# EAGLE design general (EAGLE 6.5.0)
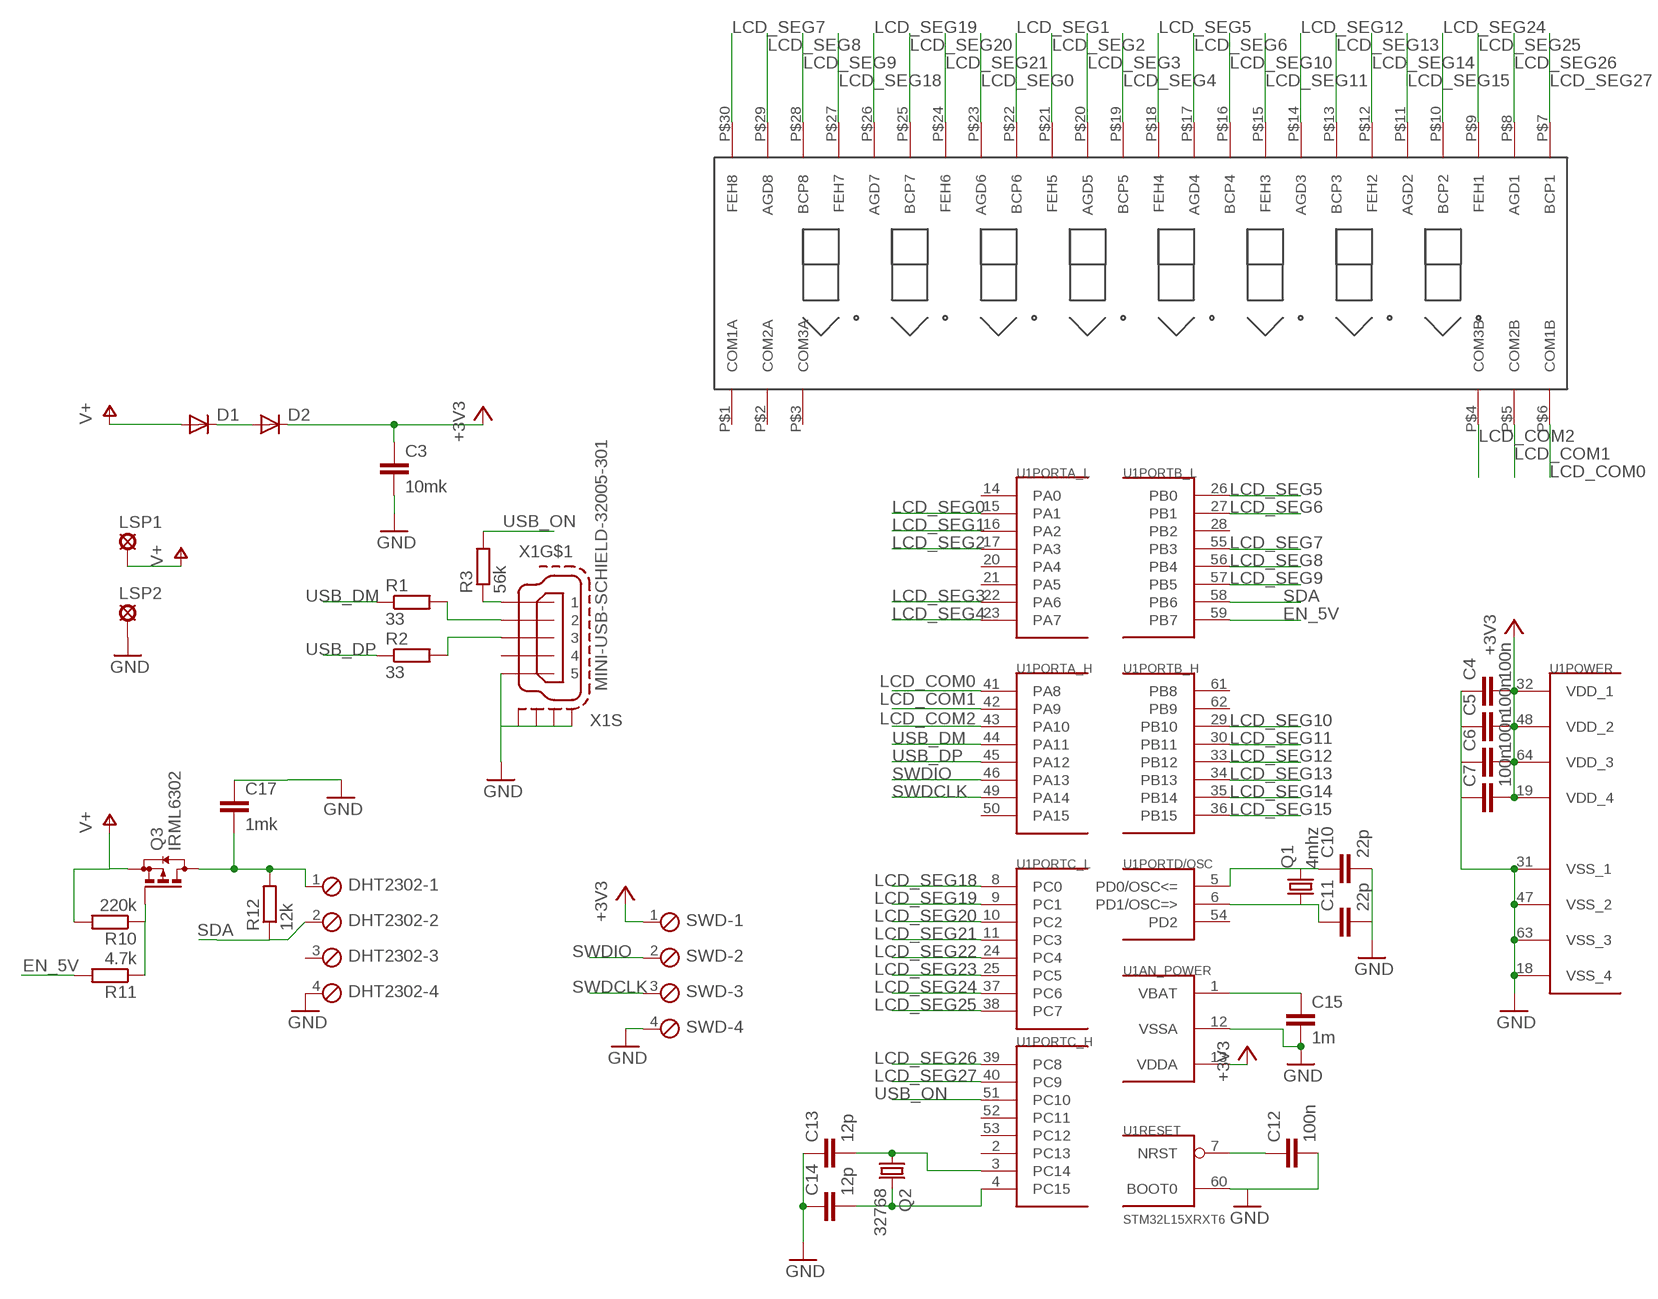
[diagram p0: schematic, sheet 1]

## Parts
C3  10mk  C-EUC0805  [C0805]
C4  100n  C-EUC0603  [C0603]
C5  100n  C-EUC0603  [C0603]
C6  100n  C-EUC0603  [C0603]
C7  100n  C-EUC0603  [C0603]
C10  22p  C-EUC0603  [C0603]
C11  22p  C-EUC0603  [C0603]
C12  100n  C-EUC0603  [C0603]
C13  12p  C-EUC0805  [C0805]
C14  12p  C-EUC0805  [C0805]
C15  1m  C-EUC0603  [C0603]
C17  1mk  C-EUC0603  [C0603]
D1  CGRM4004-G  [SOD-123_MINI-SMA]
D2  CGRM4004-G  [SOD-123_MINI-SMA]
DHT2302  MPT4  [4POL254]
LSP1  SE14  [SE14]
LSP2  SE14  [SE14]
Q1  4mhz  CRYSTALHC49S  [HC49/S]
Q2  32768  CRYSTALTC26H  [TC26H]
Q3  IRML6302  BSS84  [SOT23]
R1  33  R-EU_M0805  [M0805]
R2  33  R-EU_M0805  [M0805]
R3  56k  R-EU_R0805  [R0805]
R10  220k  R-EU_R0805  [R0805]
R11  4.7k  R-EU_R0805  [R0805]
R12  12k  R-EU_R0805  [R0805]
SWD  MPT4  [4POL254]
U1  STM32L15XRXT6  STM32F10XRXT6  [TQFP64]
U$1  TI8077  [TI8077]
X1  MINI-USB-SCHIELD-32005-301  [32005-301]

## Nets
+3V3: C3.1 C4.2 C5.2 C6.2 C7.2 D2.C SWD.1 U1.13(AN_POWER:VDDA) U1.19(POWER:VDD_4) U1.32(POWER:VDD_1) U1.48(POWER:VDD_2) U1.64(POWER:VDD_3)
+5V: D1.A LSP1.MP Q3.2(S) R10.2 ; supply symbol labelled V+
EN_5V: R11.2 U1.59(PORTB_L:PB7)
GND: C3.2 C4.1 C5.1 C6.1 C7.1 C10.2 C11.2 C12.2 C13.1 C14.1 C15.2 C17.1 DHT2302.4 LSP2.MP SWD.4 U1.12(AN_POWER:VSSA) U1.18(POWER:VSS_4) U1.31(POWER:VSS_1) U1.47(POWER:VSS_2) U1.60(RESET:BOOT0) U1.63(POWER:VSS_3) X1.5 X1.M1(S:S1) X1.M2(S:S2) X1.M3(S:S3) X1.M4(S:S4)
LCD_COM0: U1.41(PORTA_H:PA8) U$1.P$6(COM1B)
LCD_COM1: U1.42(PORTA_H:PA9) U$1.P$5(COM2B)
LCD_COM2: U1.43(PORTA_H:PA10) U$1.P$4(COM3B)
LCD_SEG0: U1.15(PORTA_L:PA1) U$1.P$23(AGD6)
LCD_SEG1: U1.16(PORTA_L:PA2) U$1.P$22(BCP6)
LCD_SEG2: U1.17(PORTA_L:PA3) U$1.P$21(FEH5)
LCD_SEG3: U1.22(PORTA_L:PA6) U$1.P$20(AGD5)
LCD_SEG4: U1.23(PORTA_L:PA7) U$1.P$19(BCP5)
LCD_SEG5: U1.26(PORTB_L:PB0) U$1.P$18(FEH4)
LCD_SEG6: U1.27(PORTB_L:PB1) U$1.P$17(AGD4)
LCD_SEG7: U1.55(PORTB_L:PB3) U$1.P$30(FEH8)
LCD_SEG8: U1.56(PORTB_L:PB4) U$1.P$29(AGD8)
LCD_SEG9: U1.57(PORTB_L:PB5) U$1.P$28(BCP8)
LCD_SEG10: U1.29(PORTB_H:PB10) U$1.P$16(BCP4)
LCD_SEG11: U1.30(PORTB_H:PB11) U$1.P$15(FEH3)
LCD_SEG12: U1.33(PORTB_H:PB12) U$1.P$14(AGD3)
LCD_SEG13: U1.34(PORTB_H:PB13) U$1.P$13(BCP3)
LCD_SEG14: U1.35(PORTB_H:PB14) U$1.P$12(FEH2)
LCD_SEG15: U1.36(PORTB_H:PB15) U$1.P$11(AGD2)
LCD_SEG18: U1.8(PORTC_L:PC0) U$1.P$27(FEH7)
LCD_SEG19: U1.9(PORTC_L:PC1) U$1.P$26(AGD7)
LCD_SEG20: U1.10(PORTC_L:PC2) U$1.P$25(BCP7)
LCD_SEG21: U1.11(PORTC_L:PC3) U$1.P$24(FEH6)
LCD_SEG22: U1.24(PORTC_L:PC4)
LCD_SEG23: U1.25(PORTC_L:PC5)
LCD_SEG24: U1.37(PORTC_L:PC6) U$1.P$10(BCP2)
LCD_SEG25: U1.38(PORTC_L:PC7) U$1.P$9(FEH1)
LCD_SEG26: U1.39(PORTC_H:PC8) U$1.P$8(AGD1)
LCD_SEG27: U1.40(PORTC_H:PC9) U$1.P$7(BCP1)
N$1: R1.2 X1.2
N$2: R2.2 X1.3
N$3: D1.C D2.A
N$9: C14.2 Q2.2 U1.4(PORTC_H:PC15)
N$10: Q3.1(G) R10.1 R11.1
N$11: R3.1 X1.1
N$13: C15.1 U1.1(AN_POWER:VBAT)
N$33: C10.1 Q1.2 U1.5(PORTD/OSC:PD0/OSC<=)
N$34: C11.1 Q1.1 U1.6(PORTD/OSC:PD1/OSC=>)
N$35: C13.2 Q2.1 U1.3(PORTC_H:PC14)
N$36: C12.1 U1.7(RESET:NRST)
SDA: DHT2302.2 R12.1 U1.58(PORTB_L:PB6)
STABILIZE_5V: C17.2 DHT2302.1 Q3.3(D) R12.2
SWDCLK: SWD.3 U1.49(PORTA_H:PA14)
SWDIO: SWD.2 U1.46(PORTA_H:PA13)
USB_DM: R1.1 U1.44(PORTA_H:PA11)
USB_DP: R2.1 U1.45(PORTA_H:PA12)
USB_ON: R3.2 U1.51(PORTC_H:PC10)
Unconnected: DHT2302.3 U1.2(PORTC_H:PC13) U1.14(PORTA_L:PA0) U1.20(PORTA_L:PA4) U1.21(PORTA_L:PA5) U1.28(PORTB_L:PB2) U1.50(PORTA_H:PA15) U1.52(PORTC_H:PC11) U1.53(PORTC_H:PC12) U1.54(PORTD/OSC:PD2) U1.61(PORTB_H:PB8) U1.62(PORTB_H:PB9) U$1.P$1(COM1A) U$1.P$2(COM2A) U$1.P$3(COM3A) X1.4

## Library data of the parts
C3-C7 C10-C12 C15 C17 = rcl:C-EU: CAPACITOR, European symbol
C13 C14 = resistor:C-EU: CAPACITOR, European symbol
D1 D2 = diode:CGRM400*-G: Molded plasitc,JEDEC SOD-123/Mini SMA
DHT2302 SWD = con-phoenix-254:MPT4: PHOENIX CONNECTOR; OC_FARNELL: unknown; OC_NEWARK: unknown
LSP1 LSP2 = solpad:SE14: SOLDER PAD
Q1 = crystal:CRYSTAL: CRYSTAL; OC_FARNELL: 1667008; OC_NEWARK: unknown
Q2 = crystal:CRYSTAL: CRYSTAL; OC_FARNELL: unknown; OC_NEWARK: unknown
Q3 = transistor-small-signal:BSS84: P-CHANNEL MOS FET
R1-R3 R10-R12 = rcl:R-EU_: RESISTOR, European symbol
U1 = stm32:STM32F10XRXT6: STM32F101/103 64pin LQFP
U$1 = balmer:TI8077: LCD Display
X1 = con-cypressindustries:MINI-USB-SCHIELD-: MINI USB-B Conector Source: www.cypressindustries.com; OC_FARNELL: unknown; OC_NEWARK: unknown

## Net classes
0 default: clearance 0.15 mm

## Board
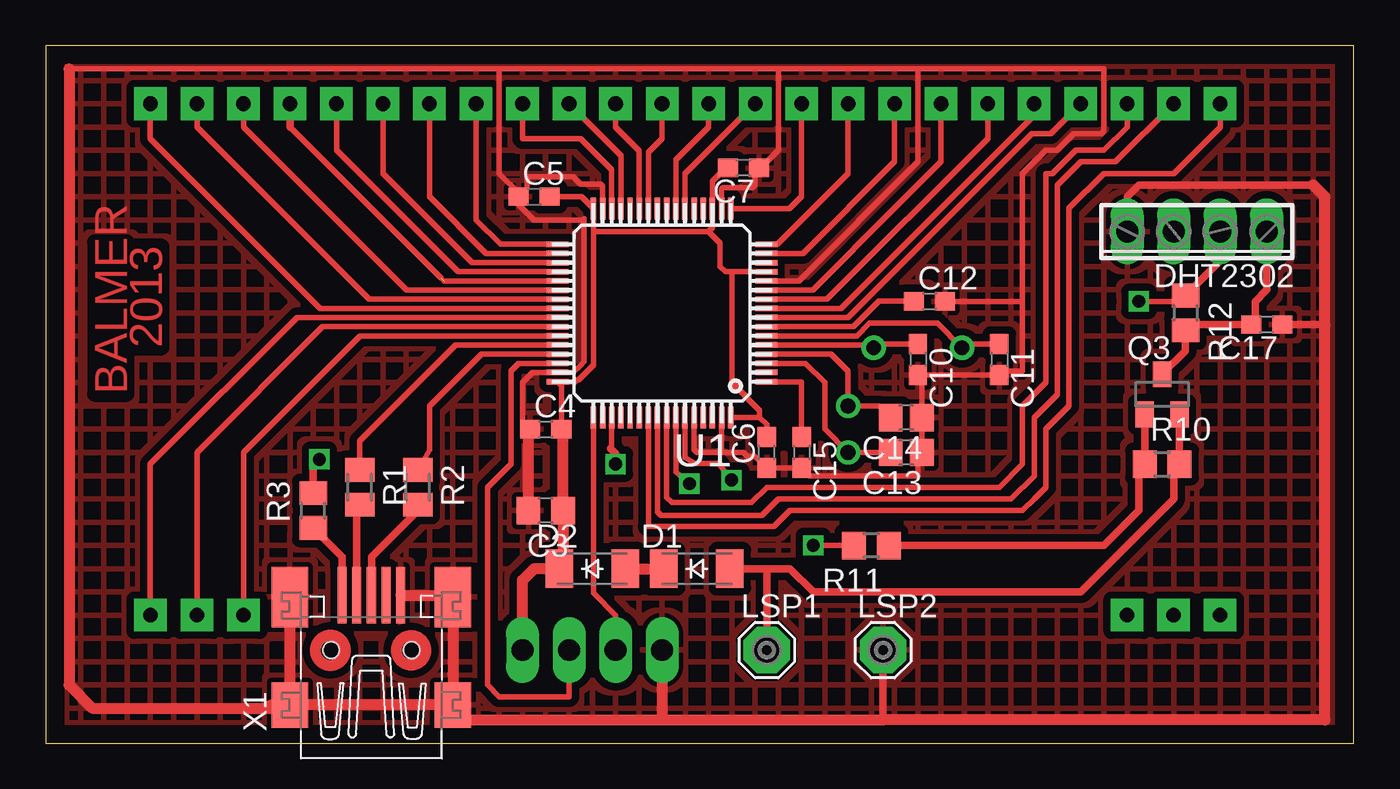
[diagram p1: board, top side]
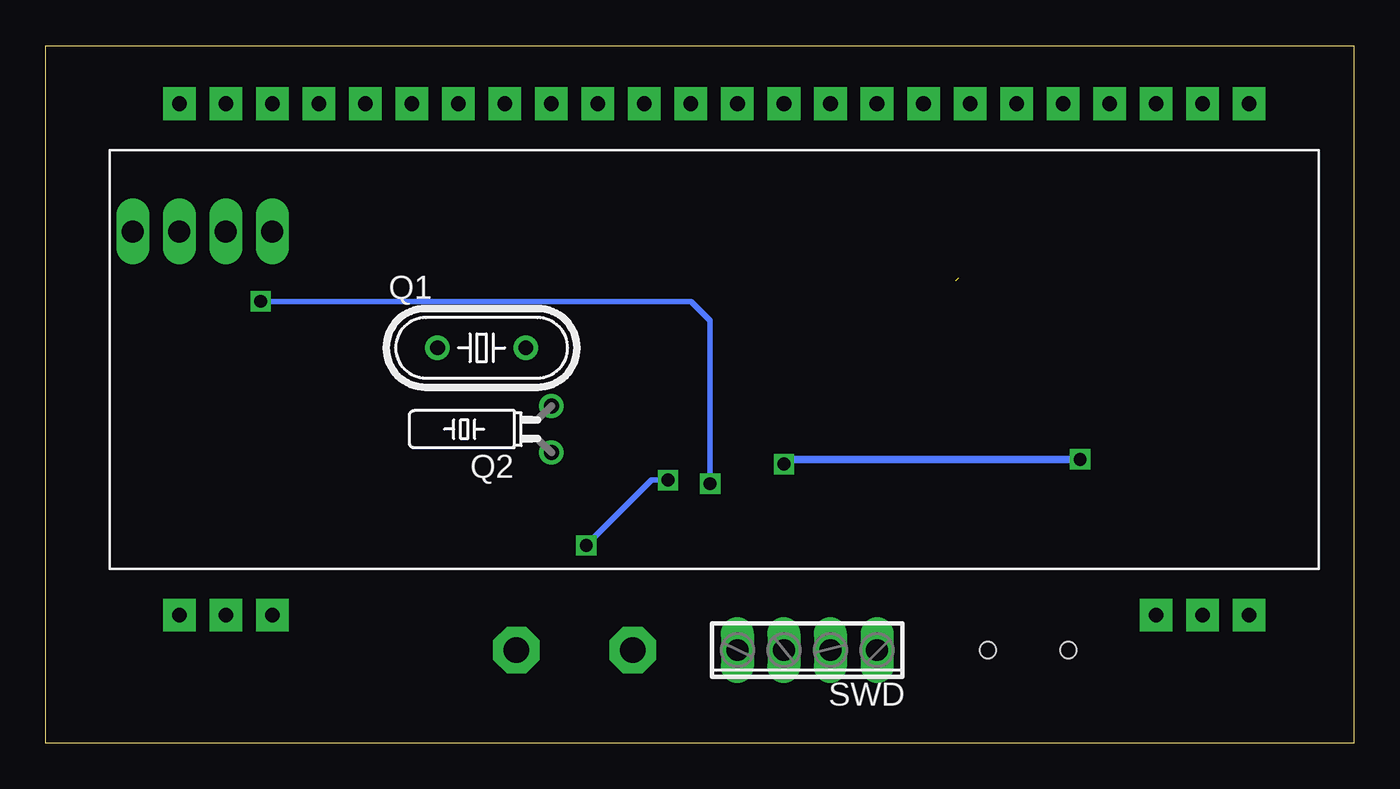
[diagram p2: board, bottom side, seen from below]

Size 71.43 x 38.09 mm. Coordinates in mm from the lower left corner, seen from the top.
Outline: 0,0 71.43,0 71.43,38.09 0,38.09 0,0
Copper layers (1*16): Top 0.035mm / dielectric 1.5mm / Bottom 0.035mm
Design rules "default": minimum track width 10mil, minimum drill 24mil, track to track 8mil, track to pad 8mil, pad to pad 8mil, via to via 8mil, smd to smd 8mil, copper to edge 40mil, drill to drill 8mil, minimum pad ring 10mil, minimum via ring 8mil, stop-mask expansion 4mil, vias tented up to drill 0mil, thermal gap 10mil

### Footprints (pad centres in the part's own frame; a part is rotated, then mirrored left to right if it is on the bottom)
C0805 = smd 1.3 x 1.5: 1 -0.95,0; 2 0.95,0
C0603 = smd 1.1 x 1: 1 -0.85,0; 2 0.85,0
C0805' = smd 1.3 x 1.5: 1 -0.85,0; 2 0.85,0
SOD-123_MINI-SMA = smd 1.5 x 2.1: A 1.8,0; C -1.8,0
4POL254 = drill 1.2 long: 1 -3.81,0; 2 -1.27,0; 3 1.27,0; 4 3.81,0
SE14 = drill 1.397 pad 2.54 octagon: MP 0,0
HC49/S = drill 0.813: 1 -2.413,0; 2 2.413,0
TC26H = drill 0.813: 1 -1.27,0; 2 1.27,0
SOT23 = smd 1 x 1.4: 1 -0.95,-1.1; 2 0.95,-1.1; 3 0,1.1
M0805 = smd 1.3 x 1.6: 1 -0.95,0; 2 0.95,0
R0805 = smd 1.3 x 1.5: 1 -0.95,0; 2 0.95,0
TQFP64 = smd 1.2 x 0.3: 1 -5.7,3.75; 2 -5.7,3.25; 3 -5.7,2.75; 4 -5.7,2.25; 5 -5.7,1.75; 6 -5.7,1.25; 7 -5.7,0.75; 8 -5.7,0.25; 9 -5.7,-0.25; 10 -5.7,-0.75; 11 -5.7,-1.25; 12 -5.7,-1.75; 13 -5.7,-2.25; 14 -5.7,-2.75; 15 -5.7,-3.25; 16 -5.7,-3.75; 33 5.7,-3.75; 34 5.7,-3.25; 35 5.7,-2.75; 36 5.7,-2.25; 37 5.7,-1.75; 38 5.7,-1.25; 39 5.7,-0.75; 40 5.7,-0.25; 41 5.7,0.25; 42 5.7,0.75; 43 5.7,1.25; 44 5.7,1.75; 45 5.7,2.25; 46 5.7,2.75; 47 5.7,3.25; 48 5.7,3.75 | smd 0.3 x 1.2: 17 -3.75,-5.7; 18 -3.25,-5.7; 19 -2.75,-5.7; 20 -2.25,-5.7; 21 -1.75,-5.7; 22 -1.25,-5.7; 23 -0.75,-5.7; 24 -0.25,-5.7; 25 0.25,-5.7; 26 0.75,-5.7; 27 1.25,-5.7; 28 1.75,-5.7; 29 2.25,-5.7; 30 2.75,-5.7; 31 3.25,-5.7; 32 3.75,-5.7; 49 3.75,5.7; 50 3.25,5.7; 51 2.75,5.7; 52 2.25,5.7; 53 1.75,5.7; 54 1.25,5.7; 55 0.75,5.7; 56 0.25,5.7; 57 -0.25,5.7; 58 -0.75,5.7; 59 -1.25,5.7; 60 -1.75,5.7; 61 -2.25,5.7; 62 -2.75,5.7; 63 -3.25,5.7; 64 -3.75,5.7
TI8077 = drill 0.8 pad 1.778 square: P$1 -27.94,-13.97; P$2 -25.4,-13.97; P$3 -22.86,-13.97; P$4 25.4,-13.97; P$5 27.94,-13.97; P$6 30.48,-13.97; P$7 30.48,13.97; P$8 27.94,13.97; P$9 25.4,13.97; P$10 22.86,13.97; P$11 20.32,13.97; P$12 17.78,13.97; P$13 15.24,13.97; P$14 12.7,13.97; P$15 10.16,13.97; P$16 7.62,13.97; P$17 5.08,13.97; P$18 2.54,13.97; P$19 0,13.97; P$20 -2.54,13.97; P$21 -5.08,13.97; P$22 -7.62,13.97; P$23 -10.16,13.97; P$24 -12.7,13.97; P$25 -15.24,13.97; P$26 -17.78,13.97; P$27 -20.32,13.97; P$28 -22.86,13.97; P$29 -25.4,13.97; P$30 -27.94,13.97
32005-301 = smd 3.1 x 0.5: 1 3,1.6; 2 3,0.8; 3 3,0; 4 3,-0.8; 5 3,-1.6 | smd 2.5 x 2: M1 -3,-4.45; M2 -3,4.45 | smd 3.3 x 2: M3 2.9,4.45; M4 2.9,-4.45 | hole 0.9: 0,2.2; 0,-2.2

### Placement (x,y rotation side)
C3  27.3,12.7 180 top
C4  27.3,17.14 0 top
C5  26.67,29.84 0 top
C6  39.37,15.88 90 top
C7  38.1,31.41 180 top
C10  47.62,20.95 270 top
C11  52.07,20.95 270 top
C12  48.26,24.13 0 top
C13  12p  [C0805']  46.99,15.88 180 top
C14  12p  [C0805']  46.99,17.78 180 top
C15  41.27,15.88 270 top
C17  66.67,22.86 180 top
D1  35.56,9.53 0 top
D2  29.84,9.53 0 top
DHT2302  62.87,27.94 180 top
LSP1  39.37,5.08 0 top
LSP2  45.72,5.08 0 top
Q1  47.62,21.59 0 bottom
Q2  43.81,17.14 90 bottom
Q3  60.96,19.05 0 top
R1  17.14,13.97 270 top
R2  20.32,13.97 270 top
R3  14.61,12.7 90 top
R10  60.96,15.24 0 top
R11  45.09,10.79 180 top
R12  62.23,23.49 270 top
SWD  29.84,5.08 180 bottom
U1  33.66,23.49 180 top
U$1  36.2,20.95 0 bottom
X1  17.78,5.08 90 top

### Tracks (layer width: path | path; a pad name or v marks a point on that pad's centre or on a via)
+3V3
  Top 0.3: C4.2 28.16,19.54 U1.48 28.89,19.73 28.99,19.83 29.09,19.83 29.91,20.65 29.91,27.94 | C5.2 29.25,29.84 U1.32 29.91,27.94 | C7.2 36.95,31.11 36.83,31.11 36.41,30.69 U1.19 36.41,28.15 36.2,27.94 | 36.2,27.94 29.91,27.94 | 37.12,25.74 36.83,26.04 36.83,27.3 36.2,27.94
  Top 0.305: U1.64 38.98,17.79 | C6.2 39.37,17.41 38.98,17.79 | U1.13 37.47,25.74 | 37.47,25.74 37.12,25.74 | 38.98,17.79 38.98,18.16 37.47,19.68 37.47,25.74
  Top 0.61: C4.2 28.25,17.04 C3.1 28.25,11.11 28.25,9.73 D2.C 26.67,9.53 26.04,8.89 SWD.1
+5V
  Top 0.406: D1.A 39.37,9.53 | 39.37,9.53 40.64,9.53 41.91,8.26 56.52,8.26 61.59,13.34 61.59,14.93 R10.2 Q3.2 | LSP1.MP 39.37,9.53
EN_5V  (via drill 0.7)
  Top 0.305: U1.59 34.91,15.6 35.45,15.27 36.74,15.27 v37.45,14.37 | v41.91,10.79 R11.2
  Bottom 0.305: v37.45,14.37 38.34,14.37 v41.91,10.79
GND
  Top 0.3: C4.1 26.04,17.56 26.04,19.68 26.59,20.24 U1.47 28.79,20.23 29.19,20.63 29.39,20.83 29.39,28.63 29.33,28.57 26.67,28.57 25.82,29.42 C5.1 25.89,29.91 | U1.60 35.41,16.03 35.56,15.88 36.83,15.88 36.91,15.95 | U1.63 36.91,15.95 | U1.31 30.41,30.42 30.29,30.54 29.19,30.54 28.79,30.93 26.91,30.93 26.29,30.93 | U1.18 36.91,29.85 36.91,30.25 36.99,30.33 38.59,30.33 38.73,30.48 38.73,31.2 | 38.73,31.2 C7.1 | 38.31,15.66 38.1,15.88 36.98,15.88 36.91,15.95 | C12.2 53.34,24.13 | 52.29,20.32 C11.2 C10.2 47.84,19.89 C14.1 C13.1 47.62,15.66 47.62,14.61 42.55,14.61 | 38.73,31.2 38.82,31.2 40.01,32.39 40.01,36.83 24.77,36.83 1.27,36.83
  Top 0.305: 42.55,14.61 41.7,14.61 C15.2 C6.1 38.73,15.66 38.31,15.66 | 25.89,29.91 25.89,29.99 24.77,31.11 24.77,36.83 | 26.29,30.93 26.29,30.31 C5.1 | U1.12 41.12,25.24 47.62,31.75 47.62,36.83 | 47.62,36.83 40.01,36.83 | 47.62,36.83 57.79,36.83 57.79,35.56 57.79,33.44 57.64,33.29 56.15,33.29 55.24,32.39 54.61,32.39 53.34,31.11 53.34,24.13 53.34,20.32 52.29,20.32
  Top 0.406: 69.22,30.48 59.69,30.48 59.05,29.84 DHT2302.4 | C17.1 69.85,22.86 | LSP2.MP 45.72,1.27
  Top 0.61: X1.M3 X1.M2 | X1.M2 12.3,2.08 | X1.M1 X1.M2 | X1.5 22.13,8.08 X1.M4 22.23,3.81 X1.M1 | 22.41,1.91 X1.M1 | C3.2 26.36,17.04 C4.1 | 1.27,36.83 1.27,3.17 2.54,1.91 13.16,1.91 X1.M2 | X1.M1 22.23,1.91 22.86,1.27 33.66,1.27 | 33.66,1.27 34.92,1.27 45.72,1.27 69.85,1.27 69.85,22.86 69.85,29.84 69.22,30.48 | SWD.4 33.66,1.27
  pour Top (isolate 0.406, hatched): 0,38.1 71.12,38.1 71.12,0 0,0
LCD_COM0
  Top 0.305: U1.41 13.72,23.24 5.71,15.24 U$1.P$6
LCD_COM1
  Top 0.305: U1.42 15.12,22.74 8.26,15.88 U$1.P$5
LCD_COM2
  Top 0.305: U1.43 17.16,22.24 10.79,15.88 U$1.P$4
LCD_SEG0
  Top 0.305: U1.15 41.35,26.74 46.35,31.75 U$1.P$23
LCD_SEG1
  Top 0.305: U1.16 39.95,27.24 43.81,31.11 U$1.P$22
LCD_SEG2
  Top 0.3: U1.17 40.62,29.19 41.27,29.84 U$1.P$21
LCD_SEG3
  Top 0.305: U1.22 34.91,31.09 U$1.P$20
LCD_SEG4
  Top 0.305: U1.23 34.41,31.86 36.2,33.66 U$1.P$19
LCD_SEG5
  Top 0.305: U1.26 32.91,32.27 33.66,33.02 U$1.P$18
LCD_SEG6
  Top 0.305: U1.27 32.41,32.37 31.12,33.66 U$1.P$17
LCD_SEG7
  Top 0.3: U1.55 32.91,12.81 | 55.88,18.41 54.61,17.14 54.61,13.97 53.98,13.34 53.34,12.7 40.64,12.7 39.77,11.84 32.89,11.84
  Top 0.305: 55.88,18.41 55.88,25.4 55.88,29.21 57.79,31.11 61.59,31.11 64.13,33.66 U$1.P$30 | 32.91,12.81 32.91,11.85 32.89,11.84
LCD_SEG8
  Top 0.3: U1.56 33.41,13.59 33.41,12.62 33.59,12.44 39.1,12.44 40.01,13.34 52.07,13.34 52.7,13.34 53.98,14.61 53.98,17.78 55.24,19.05
  Top 0.305: 55.24,19.05 55.24,26.67 55.24,30.48 56.52,31.75 58.42,31.75 U$1.P$29
LCD_SEG9
  Top 0.3: U1.57 33.91,14.36 33.91,13.42 34.19,13.13 38.54,13.13 39.37,13.97 52.07,13.97 53.34,15.24 53.34,17.78 53.34,18.41 54.61,19.68
  Top 0.305: 54.61,19.68 54.61,31.11 54.97,31.11 56.24,32.39 57.79,32.39 59.05,33.66 U$1.P$28
LCD_SEG10
  Top 0.305: U1.29 31.41,32.09 31.12,32.39 U$1.P$16
LCD_SEG11
  Top 0.305: U1.30 30.91,31.32 29.21,33.02 26.04,33.02 U$1.P$15
LCD_SEG12
  Top 0.3: U1.33 24.82,27.24 23.5,28.57 U$1.P$14
LCD_SEG13
  Top 0.3: U1.34 24.05,26.74
  Top 0.305: 24.05,26.74 20.96,29.84 U$1.P$13
LCD_SEG14
  Top 0.3: U1.35 23.29,26.24
  Top 0.305: 23.29,26.24 18.41,31.11 U$1.P$12
LCD_SEG15
  Top 0.3: U1.36 22.52,25.74
  Top 0.305: 22.52,25.74 15.88,32.39 U$1.P$11
LCD_SEG18
  Top 0.3: U1.8 43.7,23.24
  Top 0.305: 43.7,23.24 43.79,23.24 43.8,23.24 53.84,33.29 54.88,33.29 U$1.P$27
LCD_SEG19
  Top 0.3: U1.9 43.43,23.74
  Top 0.305: 43.43,23.74 53.98,34.29 U$1.P$26
LCD_SEG20
  Top 0.3: U1.10 42.66,24.24
  Top 0.305: 42.66,24.24 51.44,33.02 U$1.P$25
LCD_SEG21
  Top 0.3: U1.11 41.89,24.74 46.35,29.21 48.9,31.75 U$1.P$24
LCD_SEG24  (1 unrouted)
  Top 0.3: U1.37 21.75,25.24
  Top 0.305: 21.59,25.4 13.34,33.66
  Top 0.406: 13.34,33.66 U$1.P$10
LCD_SEG25
  Top 0.305: U1.38 19.7,24.74 10.79,33.66 U$1.P$9
LCD_SEG26
  Top 0.305: U1.39 17.66,24.24 8.26,33.66 U$1.P$8
LCD_SEG27
  Top 0.305: U1.40 14.99,23.74 5.71,33.02 U$1.P$7
N$1
  Top 0.406: X1.2 16.98,12.86 R1.2
N$2
  Top 0.406: X1.3 17.78,10.16 19.05,11.43 20.32,12.7 R2.2
N$3
  Top 0.61: D2.A D1.C
N$9
  Top 0.3: U1.4 42.89,21.24 43.81,20.32 Q2.2 45.51,18.41 C14.2
N$10
  Top 0.406: Q3.1 R10.1 59.69,14.92 59.69,12.7 57.79,10.79 R11.1
N$11
  Top 0.406: X1.1 16.18,10.18 R3.1
N$13
  Top 0.3: 39.37,19.73 U1.1
  Top 0.305: 39.37,19.73 41.23,19.73 41.27,19.68 C15.1
N$33
  Top 0.3: U1.5 45.06,21.74 Q1.2 45.43,21.8 C10.1
N$34
  Top 0.3: U1.6 44.3,22.24 44.99,22.93 48.69,22.93 Q1.1 50.25,21.8 C11.1
N$35
  Top 0.3: U1.3 41.48,20.74 42.55,19.68 42.55,17.14 Q2.1 C13.2
N$36
  Top 0.3: U1.7 44.1,22.74 45.49,24.13 C12.1
SDA  (via drill 0.7)
  Top 0.305: U1.58 34.41,14.8 v35.14,14.17 | v59.69,24.13 61.91,24.13 R12.1
  Top 0.406: DHT2302.2 64.13,26.35 R12.1
  Bottom 0.305: v35.14,14.17 35.14,23.08 36.2,24.13 v59.69,24.13
STABILIZE_5V
  Top 0.406: DHT2302.1 66.67,24.76 66.04,24.13 66.04,23.07 C17.2 62.55,22.86 R12.2 62.23,21.42 Q3.3
SWDCLK
  Top 0.305: U1.49 29.91,8.2 31.12,6.99 SWD.3
SWDIO
  Top 0.3: U1.46 25.82,20.74 25.4,20.32 25.4,15.24
  Top 0.305: 25.4,15.24 24.13,13.97 24.13,3.17 24.77,2.54 28.57,2.54 SWD.2
USB_DM
  Top 0.3: U1.44 22.38,21.74 17.78,17.14 17.14,16.51 R1.1
USB_DP
  Top 0.3: U1.45 23.79,21.24 23.5,20.95 20.96,18.41 20.96,16 R2.1
USB_ON  (via drill 0.7)
  Top 0.305: U1.51 30.91,16.16 30.84,16.1
  Top 0.406: R3.2 14.61,15.17 v14.94,15.5 | v31.12,15.24 31.12,15.83 30.84,16.1
  Bottom 0.406: v14.94,15.5 30.86,15.5 v31.12,15.24
(copper drawn outside any net)
  shapes: Top circle x2

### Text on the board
Top: 2013 | BALMER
